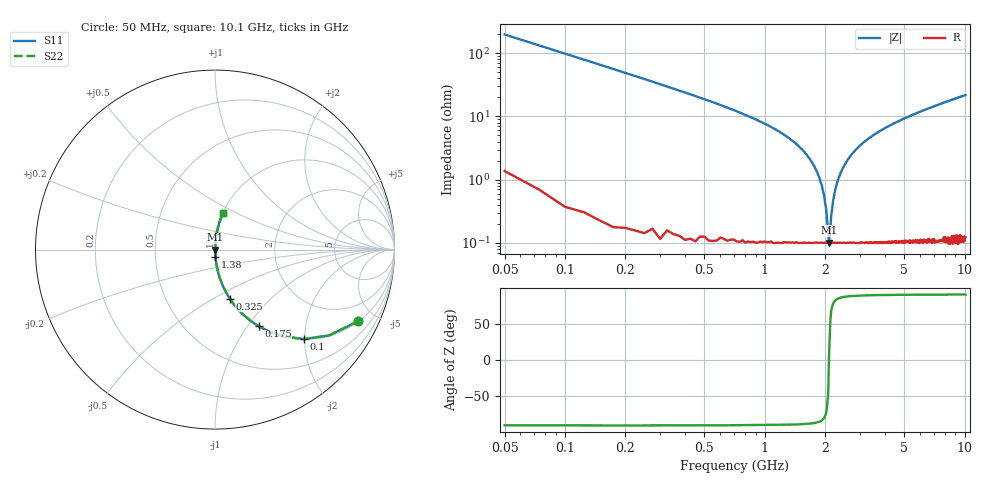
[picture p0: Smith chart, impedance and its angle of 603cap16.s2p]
! AVX Thin Film Operation		Date: November 2004
! Description: Accu-P® Series, Thin Film, SMD, RF Capacitor
! Part Number: 06033J160FBT
! 50 MHz  -  10.05 GHz
! Serial Measurements
# hz S db R 50
!	S11		S21		S12		S22
!	dB	Phase	dB	Phase	dB	Phase	dB	Phase
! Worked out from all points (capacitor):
!   400 points, 50 MHz to 10.1 GHz, reference 50 ohm
!   read as one part in series: C = 16 pF near 100 MHz
!   lowest |Z| = 101 mohm at 2.1 GHz (marker M1)
!   series resonance near 2.098 GHz, so ESL is about 360 pH
!   S11 on the Smith chart (normalised r, x): 50 MHz: 1.03, -3.98; 100 MHz: 1.01, -1.99; 175 MHz: 1.00, -1.13; 325 MHz: 1.00, -0.60; 1.38 GHz: 1.00, -0.08; 10.1 GHz: 1.00, +0.43
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5e7  -1.00 -26.6  -6.97 63.0  -6.97 63.0  -1.00 -26.6
1e8  -3.06 -45.1  -3.00 44.7  -3.00 44.7  -3.06 -45.1
1.75e8  -6.18 -60.4  -1.21 29.4  -1.21 29.4  -6.18 -60.4
3.25e8  -10.90 -73.1  -0.38 16.6  -0.38 16.6  -10.90 -73.1
7e8  -18.10 -82.3  -0.08 7.2  -0.08 7.2  -18.10 -82.3
1.38e9  -27.70 -86.2  -0.02 2.4  -0.02 2.4  -27.70 -86.2
1.73e9  -34.60 -85.9  -0.01 1.1  -0.01 1.1  -34.60 -85.9
1.88e9  -39.40 -84.0  -0.01 0.6  -0.01 0.6  -39.40 -84.0
1.98e9  -44.80 -79.7  -0.01 0.3  -0.01 0.3  -44.80 -79.7
2.03e9  -49.20 -73.0  -0.01 0.2  -0.01 0.2  -49.20 -73.0
2.1e9  -59.90 7.6  -0.01 -0.0  -0.01 -0.0  -59.90 7.6
2.13e9  -55.90 51.4  -0.01 -0.1  -0.01 -0.1  -55.90 51.4
2.15e9  -51.80 67.0  -0.01 -0.1  -0.01 -0.1  -51.80 67.0
2.2e9  -46.60 77.3  -0.01 -0.3  -0.01 -0.3  -46.60 77.3
2.3e9  -41.10 83.0  -0.01 -0.5  -0.01 -0.5  -41.10 83.0
2.4e9  -37.80 84.8  -0.01 -0.7  -0.01 -0.7  -37.80 84.8
2.8e9  -31.10 86.3  -0.01 -1.6  -0.01 -1.6  -31.10 86.3
3.4e9  -26.50 86.1  -0.02 -2.7  -0.02 -2.7  -26.50 86.1
5.08e9  -20.50 83.9  -0.05 -5.4  -0.05 -5.4  -20.50 83.9
6.75e9  -17.30 81.7  -0.09 -7.8  -0.09 -7.8  -17.30 81.7
8.43e9  -15.10 79.5  -0.15 -10.1  -0.15 -10.1  -15.10 79.5
1.01e10  -13.50 77.4  -0.21 -12.3  -0.21 -12.3  -13.50 77.4
